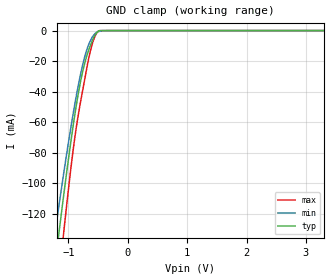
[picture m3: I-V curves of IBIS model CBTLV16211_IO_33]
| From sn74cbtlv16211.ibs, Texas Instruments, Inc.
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[Model]   CBTLV16211_IO_33
Model_type  Terminator
| variable   typ   min   max
C_comp   3.82pF   3.25pF   4.38pF
| C_tri-state   3.82pF   3.25pF   4.38pF
[Temperature Range]   40   100   -40
| Ambient temperature   25   85   -40
[Voltage range]   3.3   3   3.6
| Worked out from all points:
|   GND clamp passes 1 mA (typ) near -0.52 V on its own axis
[GND Clamp]
| CBTLV16211_IO_33
|   Voltage   I(typ)   I(min)   I(max)
-5.5V     -1.743A    -1.502A    -2.1A
-1.25V    -161.7mA   -139.7mA   -197.7mA
-1.21V    -148.8mA   -128.6mA   -182mA
-1.175V   -137.6mA   -119.1mA   -168.5mA
-1.14V    -126.6mA   -109.6mA   -155.1mA
-1.075V   -106.6mA   -92.51mA   -130.9mA
-910mV    -59.82mA   -52.25mA   -75.36mA
-775mV    -29.58mA   -25.07mA   -42.43mA
-695mV    -17.21mA   -13.22mA   -25.58mA
-620mV    -8.726mA   -5.827mA   -11.86mA
-500mV    -466.3uA   -767.1uA   -499.5uA
3.3V      1.257nA    61.35nA    15.91pA
